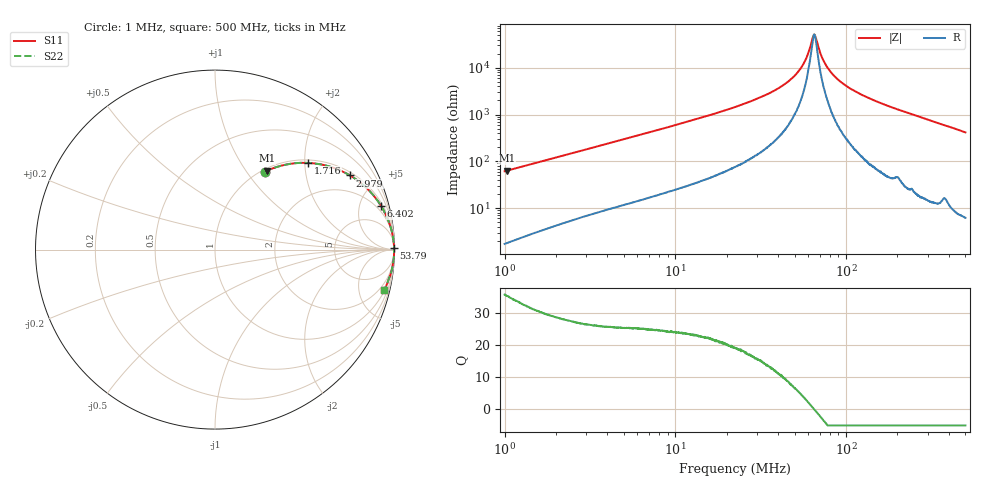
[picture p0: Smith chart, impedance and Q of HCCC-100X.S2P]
!s-Parameter Generated by FASTRON Sdn. Bhd.
!FASTRON P/N : HCCC-100X
!Keysight Technologies,E4991B,MY54100416,A.01.15
!Date: Mon Apr 06 14:07:55 2026
!Version  : Rev00 Mon Apr 06 14:07:55 2026
!Data & Calibration Information:
!PortZ  Port1:50+j0  Port2:50+j0
!When reading, reference impedance value at option line is always used.
! Remarks : This data is being provided solely for informational purposes.
!Freq	S11	S21	S12	S22
# Hz S dB R 50
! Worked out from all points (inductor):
!   1601 points, 1 MHz to 500 MHz, reference 50 ohm
!   read as one part in series: L = 9.67 uH near 1.032 MHz
!   highest Q = 35.3 at 1.032 MHz (marker M1), where L = 9.71 uH
!   self-resonance near 65.07 MHz
!   S11 on the Smith chart (normalised r, x): 1 MHz: 1.03, +1.22; 1.716 MHz: 1.07, +2.07; 2.979 MHz: 1.13, +3.56; 6.402 MHz: 1.30, +7.55; 53.79 MHz: open; 500 MHz: 1.12, -8.30
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1000000  -5.77 57.4  -1.48 -31.0  -1.48 -31.0  -5.77 57.4
1031561  -5.58 56.6  -1.56 -31.7  -1.56 -31.7  -5.58 56.6
1715825  -3.00 43.0  -3.32 -45.1  -3.32 -45.1  -3.00 43.0
2820919  -1.45 30.1  -5.99 -57.8  -5.99 -57.8  -1.45 30.1
2978562  -1.33 28.8  -6.34 -59.0  -6.34 -59.0  -1.33 28.8
6402024  -0.38 14.7  -11.92 -73.1  -11.92 -73.1  -0.38 14.7
7957584  -0.26 11.9  -13.70 -75.8  -13.70 -75.8  -0.26 11.9
2.236068e7  -0.05 3.9  -23.24 -83.1  -23.24 -83.1  -0.05 3.9
3.942448e7  -0.03 1.6  -30.90 -83.4  -30.90 -83.4  -0.03 1.6
4.713694e7  -0.02 1.0  -34.86 -81.7  -34.86 -81.7  -0.02 1.0
5.379161e7  -0.02 0.6  -39.39 -78.0  -39.39 -78.0  -0.02 0.6
5.859025e7  -0.02 0.3  -44.16 -70.1  -44.16 -70.1  -0.02 0.3
6.307767e7  -0.02 0.1  -51.55 -41.4  -51.55 -41.4  -0.02 0.1
6.456494e7  -0.02 0.0  -53.90 -13.0  -53.90 -13.0  -0.02 0.0
6.608728e7  -0.02 -0.0  -53.52 21.7  -53.52 21.7  -0.02 -0.0
7.142578e7  -0.02 -0.3  -45.37 68.3  -45.37 68.3  -0.02 -0.3
7.571081e7  -0.02 -0.5  -41.51 75.8  -41.51 75.8  -0.02 -0.5
8.214513e7  -0.02 -0.7  -37.79 81.0  -37.79 81.0  -0.02 -0.7
9.158278e7  -0.02 -1.1  -34.40 83.5  -34.40 83.5  -0.02 -1.1
1.18344e8  -0.02 -2.0  -29.14 85.1  -29.14 85.1  -0.02 -2.0
1.77937e8  -0.04 -3.8  -23.60 84.4  -23.60 84.4  -0.04 -3.8
5e8  -0.27 -13.5  -12.63 75.6  -12.63 75.6  -0.27 -13.5
